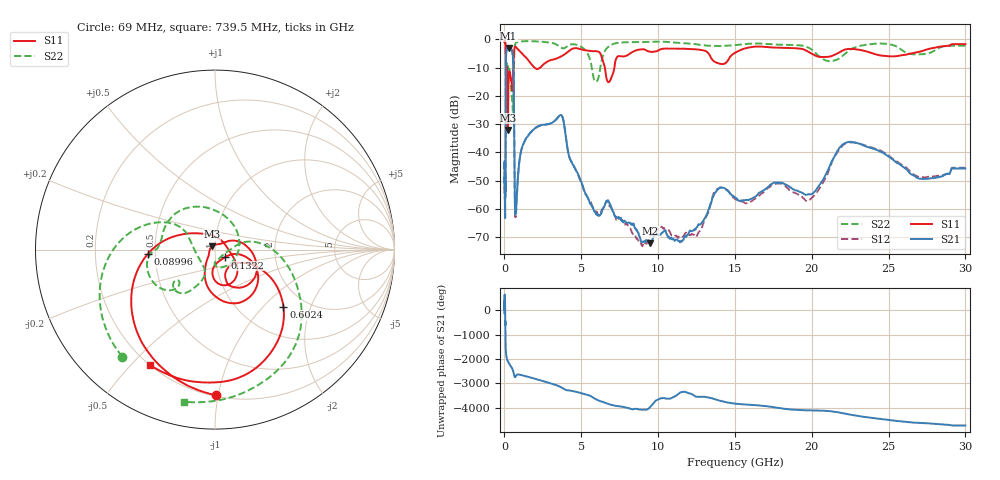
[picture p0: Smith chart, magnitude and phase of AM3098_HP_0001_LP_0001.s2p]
! Date/Time: Thu, Feb 28, 2019 8:31 AM
! Network Analyzer: Agilent Technologies E8364B Rev: A.07.50.67
! Sweep from 0.010 to 30.000 GHz, 1601 Points, Sweep Type: LOG
! Power Supply: 5.023 V, 0.002 A
# Hz S DB R 50
!freq MagS11 AngS11 MagS21 AngS21 MagS12 AngS12 MagS22 AngS22
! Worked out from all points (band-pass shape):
!   1601 points, 10 MHz to 30 GHz, reference 50 ohm
!   highest |S21| = -2.98 dB at 267.8 MHz (marker M1); lowest = -72.2 dB at 9.49 GHz (marker M2)
!   |S21| within 3 dB of the highest: 104.7 MHz to 546.1 MHz (441.4 MHz wide, 136 % of centre)
!   lowest |S11| = -32.0 dB at 227 MHz (marker M3), VSWR 1.05, Z = 48.4 + j1.84 ohm
!   |S11| at or under -10 dB: 175.6 MHz to 571.1 MHz (395.5 MHz wide, 106 % of centre); 1.964 GHz to 2.328 GHz (363.6 MHz wide, 16.9 % of centre); 6.535 GHz to 7.151 GHz (616.4 MHz wide, 9.01 % of centre)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
!   |S22| runs from -25.8 to -0.5 dB; largest |S21 - S12| = 0.013
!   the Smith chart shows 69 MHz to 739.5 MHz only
!   S11 on the Smith chart (normalised r, x): 69 MHz: 0.21, -0.99; 89.96 MHz: 0.45, -0.03; 132.2 MHz: 1.11, -0.10; 602.4 MHz: 1.55, -1.32; 739.5 MHz: 0.20, -0.57
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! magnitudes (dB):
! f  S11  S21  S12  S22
! 10 MHz  -0.4  -45.4  -43.6  -0.5
! 38.04 MHz  -0.5  -59.4  -59.1  -0.8
! 69 MHz  -1.8  -50.9  -50.3  -2.1
! 89.96 MHz  -8.5  -18.0  -18.0  -10.5
! 132.2 MHz  -23.2  -3.8  -3.8  -11.5
! 144.7 MHz  -13.4  -3.5  -3.5  -10.2
! 187.7 MHz  -11.7  -3.4  -3.4  -8.3
! 227 MHz  -32.0  -3.1  -3.0  -9.9
! 267.8 MHz  -14.7  -3.0  -3.0  -10.4
! 550.5 MHz  -13.5  -6.3  -6.2  -25.8
! 602.4 MHz  -6.1  -14.4  -14.4  -12.3
! 679.2 MHz  -2.6  -58.6  -57.9  -2.2
! 739.5 MHz  -2.6  -60.8  -61.8  -1.3
! 1.05 GHz  -4.5  -40.4  -40.5  -0.7
! 2.084 GHz  -10.5  -31.1  -31.0  -0.7
! 3.704 GHz  -6.0  -26.8  -26.9  -2.9
! 5.959 GHz  -4.2  -61.9  -60.9  -15.0
! 7.926 GHz  -5.8  -64.8  -65.4  -1.0
! 9.49 GHz  -4.4  -72.2  -69.8  -0.9
! 19.8 GHz  -4.5  -54.8  -57.0  -3.0
! 22.56 GHz  -3.4  -36.3  -36.5  -3.5
! 30 GHz  -1.7  -45.7  -45.5  -2.2
